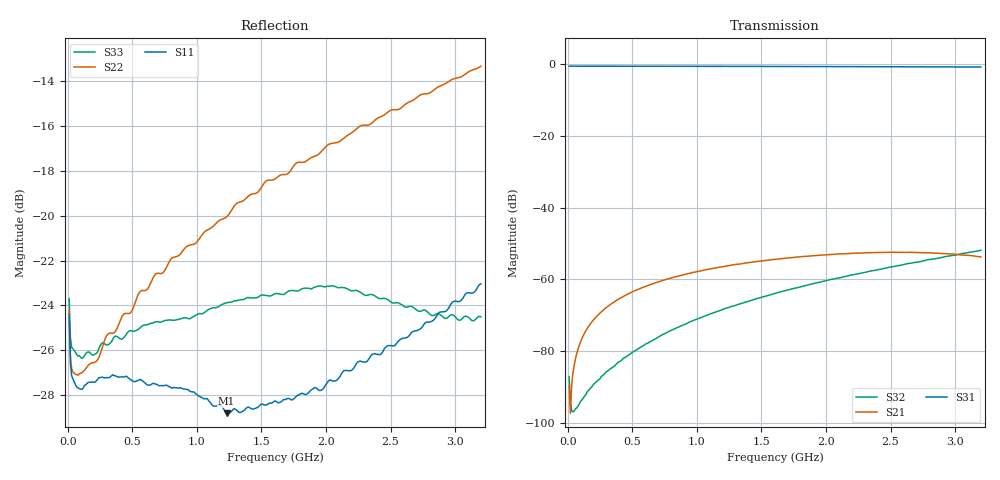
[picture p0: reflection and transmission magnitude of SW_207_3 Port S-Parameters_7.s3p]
! Created _Nov-02-2022_09-58-32
! Type : General
! Retest Level : 0
! Program : FASTESt Rev. 859
! DUT_TempC = 25.0
! Set_V1_Supply_V = 0.0
! V1_Supply_V = -0.0001
! V1_Supply_I = -3e-06
! Set_V2_Supply_V = 3.0
! V2_Supply_V = 3.0007
! V2_Supply_I = -4e-06
! RunID = 7
! SN = 4
! Comment = SW-207_SB4_RFc-RF2_room
! Input_Power = 5.0
! Measurement_Comment = None
! Freq	S11db	S11deg	S12db	S12deg	S13db	S13deg	S21db	S21deg	S22db	S22deg	S23db	S23deg	S31db	S31deg	S32db	S32deg	S33db	S33deg
# Hz S dB R 50
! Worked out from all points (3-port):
!   320 points, 10 MHz to 3.2 GHz, reference 50 ohm
!   strongest paths, dB at 10 MHz, 810 MHz, 1.61 GHz, 2.41 GHz, 3.2 GHz:
!     S31: -0.6, -0.6, -0.7, -0.7, -0.8
!     S21: -89.9, -59.6, -54.4, -52.5, -53.8
!     S32: -87.1, -74.1, -63.9, -57.3, -51.9
!   lowest |S11| = -28.8 dB at 1.23 GHz (marker M1), VSWR 1.08, Z = 47.9 - j2.86 ohm
!   |S11| at or under -10 dB: start of sweep to end of sweep
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1e7  -24.41 -43.4  -89.61 -120.7  -0.60 1.3
     -89.87 -122.4  -24.24 -38.5  -87.26 -112.6
     -0.59 1.3  -87.15 -111.7  -23.69 -40.2
7e7  -27.66 -14.7  -80.67 79.8  -0.60 -6.0
     -80.58 80.0  -27.08 -5.6  -95.40 -92.1
     -0.60 -6.0  -95.87 -94.8  -26.20 -13.2
2e8  -27.43 -16.3  -71.31 70.9  -0.61 -17.6
     -71.29 70.9  -26.55 3.7  -89.00 -129.3
     -0.61 -17.6  -89.29 -129.9  -26.21 -16.1
4.3e8  -27.19 -32.6  -64.79 53.1  -0.62 -37.7
       -64.78 53.1  -24.40 1.4  -81.96 -167.5
       -0.61 -37.7  -82.08 -168.1  -25.45 -33.4
8.5e8  -27.69 -76.2  -59.14 19.2  -0.64 -74.1
       -59.15 19.4  -21.80 -16.0  -73.38 141.7
       -0.62 -74.1  -73.44 141.6  -24.63 -74.9
1.23e9  -28.82 -124.7  -56.33 -11.2  -0.66 -107.0
        -56.27 -11.4  -20.05 -43.7  -68.01 105.3
        -0.64 -107.1  -68.06 105.0  -23.88 -115.2
1.61e9  -28.27 179.5  -54.45 -41.8  -0.68 -139.8
        -54.45 -41.9  -18.34 -73.2  -63.90 73.4
        -0.67 -139.9  -63.91 73.3  -23.47 -157.8
2.32e9  -26.49 89.4  -52.67 -99.9  -0.75 158.9
        -52.66 -99.9  -15.95 -135.1  -57.93 18.4
        -0.73 158.7  -57.95 18.3  -23.54 129.9
2.78e9  -24.75 44.3  -52.63 -137.3  -0.80 119.1
        -52.63 -137.4  -14.55 -177.3  -54.66 -15.0
        -0.78 118.9  -54.66 -15.2  -24.26 80.3
3.2e9  -23.04 3.6  -53.83 -170.8  -0.85 82.7
       -53.79 -171.0  -13.32 143.2  -51.93 -44.4
       -0.83 82.5  -51.93 -44.7  -24.51 28.2
